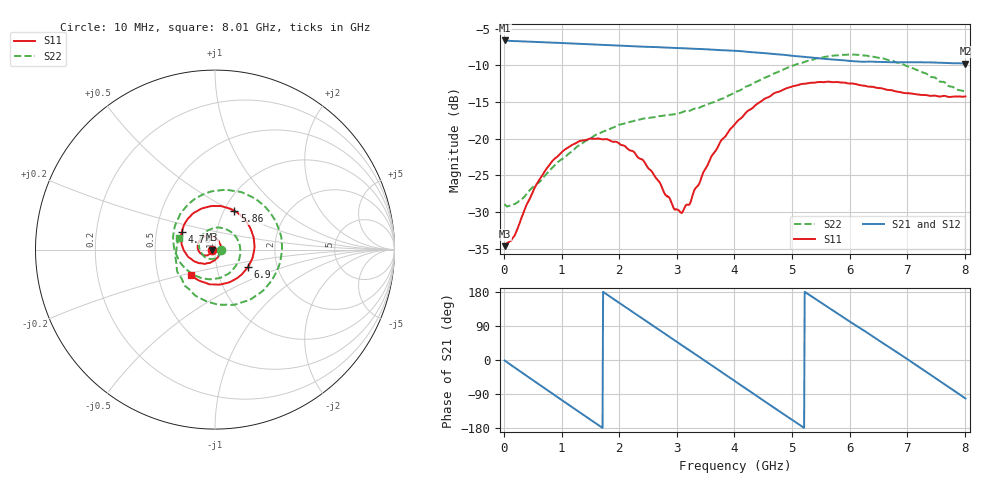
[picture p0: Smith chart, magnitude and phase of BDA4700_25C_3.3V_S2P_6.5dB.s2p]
!Agilent Technologies,E5071B,MY42404982,A.09.10
!Date: Mon Oct 20 18:05:43 2025
!Data & Calibration Information:
!Freq	S11:SOLT2(ON)	S21:SOLT2(ON)	S12:SOLT2(ON)	S22:SOLT2(ON)
# Hz S RI R 50
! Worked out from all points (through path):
!   801 points, 10 MHz to 8.01 GHz, reference 50 ohm
!   highest |S21| = -6.61 dB at 10 MHz (marker M1); lowest = -9.8 dB at 8.01 GHz (marker M2)
!   group delay of S21, straight-line fit = 284 ps
!   lowest |S11| = -34.7 dB at 10 MHz (marker M3), VSWR 1.04, Z = 48.2 - j0.0932 ohm
!   |S11| at or under -10 dB: start of sweep to end of sweep
!   |S22| runs from -29.3 to -8.5 dB; largest |S21 - S12| = 0.0054
!   S11 on the Smith chart (normalised r, x): 10 MHz: 0.96, -0.00; 4.78 GHz: 0.68, +0.14; 5.86 GHz: 1.12, +0.51; 6.9 GHz: 1.41, -0.29; 8.01 GHz: 0.74, -0.22
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1e7  -0.0185 -0.000967  0.4669 -0.0103  0.4669 -0.0104  0.0358 -0.00273
1.7e8  -0.0191 -0.00978  0.4393 -0.1456  0.4389 -0.1455  0.0317 -0.0165
3.3e8  -0.0239 -0.0195  0.3756 -0.2655  0.3754 -0.2656  0.0233 -0.0317
7.1e8  -0.0501 -0.0329  0.1164 -0.4383  0.1162 -0.4385  -0.0194 -0.0526
1.02e9  -0.079 -0.0224  -0.1346 -0.4274  -0.1346 -0.4273  -0.0645 -0.0342
1.35e9  -0.0966 0.00919  -0.3481 -0.2732  -0.3481 -0.2733  -0.0888 0.0254
1.64e9  -0.0901 0.0439  -0.4327 -0.0612  -0.4329 -0.0613  -0.066 0.0855
1.93e9  -0.0646 0.0701  -0.4005 0.1617  -0.4007 0.1616  -0.00122 0.1206
2.32e9  -0.0165 0.073  -0.1989 0.3758  -0.1988 0.3758  0.0985 0.0909
2.68e9  0.0216 0.0468  0.0665 0.4148  0.0657 0.4145  0.1416 -0.00689
3.09e9  0.0299 -0.00935  0.3232 0.2581  0.3209 0.2601  0.0889 -0.1224
3.53e9  -0.0113 -0.0645  0.4035 -0.0453  0.4036 -0.046  -0.0497 -0.1634
4.01e9  -0.1048 -0.0697  0.2223 -0.329  0.2226 -0.3279  -0.1935 -0.072
4.39e9  -0.172 -0.00756  -0.0344 -0.3849  -0.0345 -0.3858  -0.2331 0.0763
4.78e9  -0.1842 0.0997  -0.2669 -0.2633  -0.2651 -0.2649  -0.1631 0.2374
5.35e9  -0.0653 0.2314  -0.3471 0.0823  -0.3474 0.0803  0.1083 0.3264
5.86e9  0.1082 0.2157  -0.1484 0.3089  -0.1478 0.3084  0.3363 0.1605
6.25e9  0.199 0.1154  0.0718 0.3266  0.0769 0.3251  0.3631 -0.0654
6.68e9  0.2123 -0.0315  0.274 0.1877  0.2748 0.1871  0.2223 -0.2613
6.9e9  0.1816 -0.0985  0.3234 0.0719  0.3233 0.0698  0.1079 -0.3065
7.47e9  0.0258 -0.1949  0.2307 -0.2361  0.2301 -0.2367  -0.1691 -0.2002
8.01e9  -0.1321 -0.1422  -0.0652 -0.3184  -0.0645 -0.3186  -0.2 0.0644
